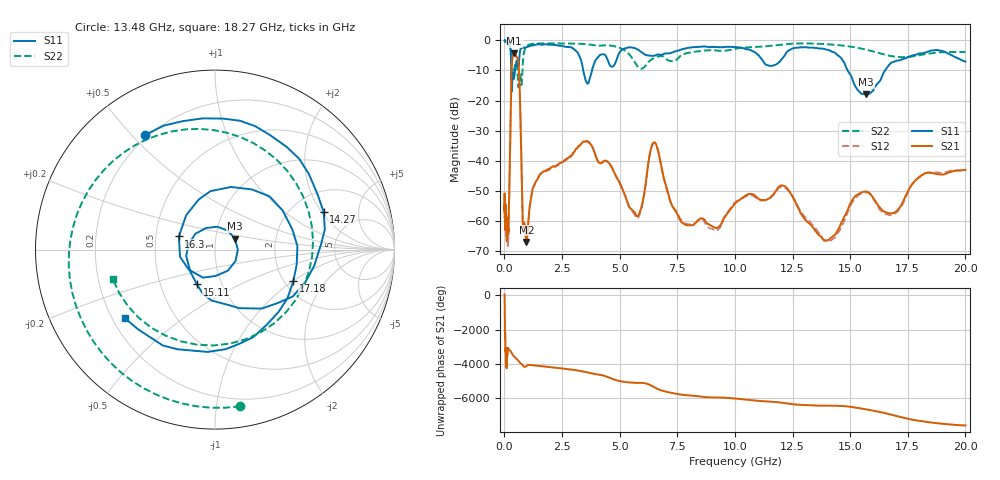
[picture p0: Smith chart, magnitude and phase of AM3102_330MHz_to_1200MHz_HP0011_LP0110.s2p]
! Date/Time: Tue, Sep 11, 2018 5:11 PM
! Network Analyzer: Agilent Technologies E8362B Rev: A.07.50.63
! Sweep from 0.010 to 20.000 GHz, 1601 Points, Sweep Type: LOG
! Power Supply: 4.950 V, 0.001 A
# Hz S DB R 50
!freq MagS11 AngS11 MagS21 AngS21 MagS12 AngS12 MagS22 AngS22
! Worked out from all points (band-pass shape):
!   1601 points, 10 MHz to 20 GHz, reference 50 ohm
!   highest |S21| = -4.31 dB at 420.4 MHz (marker M1); lowest = -67.1 dB at 956.4 MHz (marker M2)
!   |S21| within 3 dB of the highest: 328.4 MHz to 608.8 MHz (280.5 MHz wide, 59.9 % of centre)
!   lowest |S11| = -18.0 dB at 15.7 GHz (marker M3), VSWR 1.29, Z = 61.9 + j7.6 ohm
!   |S11| at or under -10 dB: 298.5 MHz to 461.9 MHz (163.4 MHz wide, 43 % of centre); 3.421 GHz to 3.799 GHz (378.8 MHz wide, 10.5 % of centre); 14.89 GHz to 16.51 GHz (1.623 GHz wide, 10.3 % of centre)
!   |S22| runs from -15.6 to -0.2 dB; largest |S21 - S12| = 0.01
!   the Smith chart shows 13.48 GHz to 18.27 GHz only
!   S11 on the Smith chart (normalised r, x): 13.48 GHz: 0.19, +0.55; 14.27 GHz: 2.96, +2.10; 15.11 GHz: 0.76, -0.31; 16.3 GHz: 0.66, +0.10; 17.18 GHz: 2.24, -1.01; 18.27 GHz: 0.25, -0.32
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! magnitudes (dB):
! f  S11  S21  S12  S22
! 10 MHz  0.0  -53.3  -50.8  -0.2
! 35.55 MHz  0.0  -61.5  -61.5  -0.4
! 126.4 MHz  -0.4  -62.9  -64.0  -0.9
! 172.9 MHz  -0.8  -63.1  -65.4  -1.1
! 420.4 MHz  -12.6  -4.3  -4.4  -10.0
! 447.2 MHz  -10.8  -4.4  -4.5  -8.7
! 626.6 MHz  -7.6  -9.1  -9.1  -14.8
! 798.4 MHz  -2.5  -60.5  -61.0  -7.8
! 956.4 MHz  -2.3  -67.1  -66.7  -2.0
! 1.59 GHz  -1.4  -44.2  -44.3  -1.0
! 3.617 GHz  -14.4  -33.7  -33.6  -1.3
! 5.652 GHz  -2.5  -57.2  -58.0  -7.2
! 6.518 GHz  -5.1  -33.9  -34.1  -5.7
! 7.845 GHz  -2.7  -61.4  -61.0  -4.4
! 13.48 GHz  -2.5  -63.3  -62.3  -1.1
! 14.27 GHz  -3.9  -65.1  -66.0  -1.4
! 15.11 GHz  -13.2  -52.9  -53.7  -2.2
! 15.7 GHz  -18.0  -50.3  -50.6  -3.1
! 16.3 GHz  -13.4  -55.8  -56.5  -4.3
! 17.18 GHz  -6.5  -55.3  -55.9  -5.6
! 18.27 GHz  -4.0  -44.2  -44.2  -4.5
! 20 GHz  -7.1  -43.1  -43.5  -3.8
